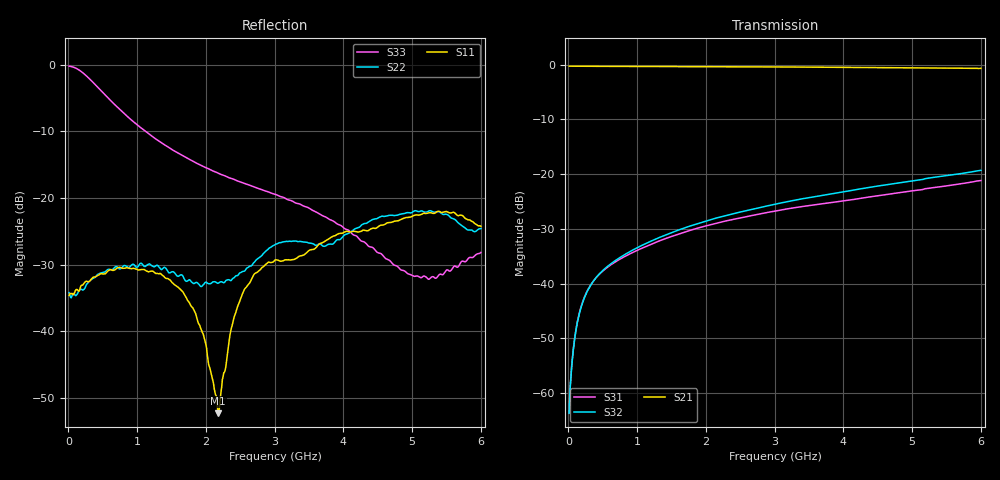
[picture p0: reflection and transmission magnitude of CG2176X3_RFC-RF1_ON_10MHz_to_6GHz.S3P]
!CEL
!CG2176X3
!Port1: RFC Port2: RF1  Port3: RF2
!Freq	S11 S12	S13 S21 S22 S23 S31 S32 S33
# Hz S dB R 50
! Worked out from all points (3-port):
!   600 points, 10 MHz to 6 GHz, reference 50 ohm
!   strongest paths, dB at 10 MHz, 1.51 GHz, 3.01 GHz, 4.51 GHz, 6 GHz:
!     S21: -0.3, -0.4, -0.4, -0.5, -0.7
!     S32: -63.7, -30.6, -25.5, -22.2, -19.3
!     S31: -63.5, -31.3, -26.7, -23.9, -21.2
!   lowest |S11| = -52.3 dB at 2.18 GHz (marker M1), VSWR 1.00, Z = 49.9 + j0.234 ohm
!   |S11| at or under -10 dB: start of sweep to end of sweep
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1e7  -34.61 -1.3  -0.28 -0.2  -63.48 47.3
     -0.28 -0.2  -34.18 -4.8  -63.78 47.9
     -63.50 48.9  -63.70 47.7  -0.20 -1.7
1.4e8  -33.87 22.3  -0.29 -1.4  -46.35 73.2
       -0.29 -1.4  -34.17 20.5  -46.53 74.6
       -46.37 73.2  -46.53 74.7  -0.68 -19.3
4e8  -31.77 37.3  -0.30 -3.7  -38.94 64.3
     -0.30 -3.7  -31.77 43.1  -38.95 67.7
     -38.95 64.3  -38.94 68.0  -3.08 -46.7
1.64e9  -33.82 38.4  -0.36 -14.2  -30.77 60.9
        -0.36 -14.2  -31.50 28.1  -30.03 66.4
        -30.80 60.7  -30.04 66.2  -13.51 -94.3
1.96e9  -40.36 33.1  -0.37 -16.9  -29.57 60.3
        -0.37 -16.9  -33.01 -1.5  -28.73 65.9
        -29.59 60.2  -28.72 65.8  -15.25 -101.1
2.18e9  -52.29 105.2  -0.38 -18.8  -28.87 59.6
        -0.38 -18.8  -32.76 -18.3  -27.93 65.2
        -28.88 59.5  -27.92 65.3  -16.26 -105.2
2.53e9  -34.40 -168.6  -0.40 -21.7  -27.89 57.9
        -0.40 -21.7  -31.04 -45.4  -26.80 64.1
        -27.93 57.9  -26.84 64.3  -17.67 -110.8
3.01e9  -29.26 -166.7  -0.43 -25.8  -26.72 55.8
        -0.42 -25.9  -26.95 -56.3  -25.45 62.4
        -26.75 55.5  -25.49 62.2  -19.43 -116.8
5.02e9  -22.62 91.7  -0.59 -43.6  -23.00 45.9
        -0.60 -43.6  -21.98 6.2  -21.15 53.8
        -23.03 45.8  -21.19 54.1  -31.69 -171.7
6e9  -24.23 94.2  -0.68 -52.4  -21.15 35.9
     -0.68 -52.5  -24.57 -12.9  -19.32 48.3
     -21.17 35.9  -19.30 47.1  -28.15 113.9
